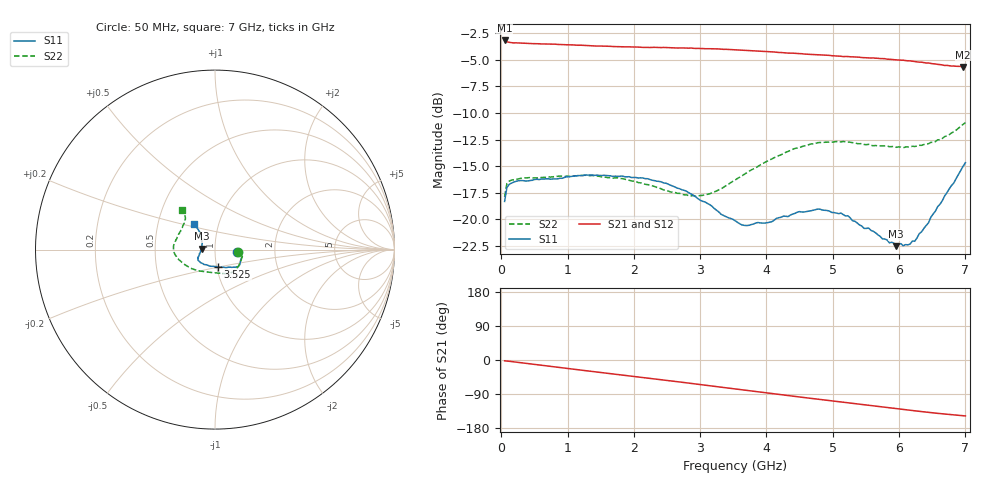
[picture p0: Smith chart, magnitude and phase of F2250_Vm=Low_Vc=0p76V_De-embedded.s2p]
! Integrated Device Technology
! Corporate Headquarters
! 6024 Silver Creek Valley Road
! San Jose, CA 95138  USA
! Phone:  1-408-284-8200
! Toll Free:  1-800-223-1366
! Webpage:  http://www.idt.com/
! Timing and RF Division
! 515 Groton Road, Suite 102
! Westford, MA 01886-6024
! Device:  F2250
! Description: Voltage Variable RF Attenuator
! Frequency:  50.0 -  6000.00 MHz
! Package:  3x3 mm Thin QFN Plastic Package: 16 pin
! Ports:  2 RF, 3 DC
!  Pin  1  = GND
!  Pin  2  = NC
!  Pin  3  = RF1  = Port 1
!  Pin  4  = NC
!  Pin  5  = GND
!  Pin  6  = GND
!  Pin  7  = GND
!  Pin  8  = GND
!  Pin  9  = NC
!  Pin 10  = RF2  = Port 2
!  Pin 11  = NC
!  Pin 12  = GND
!  Pin 13  = GND
!  Pin 14  = VCNTRL
!  Pin 15  = VDD
!  Pin 16  = VMODE
! Vcntrl:  0.760 Volts
! Vmode:  +0.000 Volts
! Vdd:  +3.30  Volts
! Current:  1.159 mA
! Data:  The device was measured on a the F2250 evaluation board which has
!  individual transmission lines to the RF pins.  Data was collected
!  using a calibrated network analyzer.  The evaluation board was
!  de-embedded using a TRL calibration technique.
!  The reference plane is the edge of the package pin.
! Misc:  SN 10
!  Action Tracker AT0258
! Date Measured:  2014-11-26
! Date:  2015-10-15  MJV
! Note:
!  Integrated Device Technology supplies this data as a sample of measured
!  data at the package pin for this product.  Your particular data for this
!  product may vary.
!  Data was taken at 25 degrees C.
!  Integrated Device Technology reserves the right to change this data at anytime.
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# GHz S dB R 50
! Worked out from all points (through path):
!   201 points, 50 MHz to 7 GHz, reference 50 ohm
!   highest |S21| = -3.17 dB at 50 MHz (marker M1); lowest = -5.7 dB at 6.965 GHz (marker M2)
!   group delay of S21, straight-line fit = 59.2 ps
!   lowest |S11| = -22.5 dB at 5.957 GHz (marker M3), VSWR 1.16, Z = 43.1 + j0.442 ohm
!   |S11| at or under -10 dB: start of sweep to end of sweep
!   |S22| runs from -17.9 to -10.9 dB; largest |S21 - S12| = 0.0019
!   S11 on the Smith chart (normalised r, x): 50 MHz: 1.27, -0.03; 3.525 GHz: 1.01, -0.20; 7 GHz: 0.76, +0.23
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0.05  -18.32 -5.0  -3.17 -2.2  -3.17 -2.2  -17.88 -6.2
0.08475  -17.01 -4.3  -3.30 -2.7  -3.30 -2.7  -16.63 -5.3
0.22375  -16.43 -7.2  -3.40 -5.6  -3.39 -5.6  -16.23 -9.7
0.77975  -16.20 -21.4  -3.51 -17.6  -3.51 -17.6  -16.01 -29.9
1.2315  -15.87 -31.3  -3.63 -27.3  -3.64 -27.3  -15.88 -45.0
1.75275  -15.96 -37.2  -3.75 -38.2  -3.75 -38.2  -16.09 -56.9
2.37825  -16.44 -40.6  -3.83 -51.2  -3.83 -51.2  -17.05 -71.3
2.93425  -17.90 -50.1  -3.92 -63.3  -3.91 -63.3  -17.82 -95.9
3.14275  -18.62 -58.8  -3.94 -67.9  -3.95 -67.9  -17.60 -108.8
3.3165  -19.54 -67.7  -3.99 -71.7  -3.99 -71.7  -17.13 -119.1
3.525  -20.13 -81.0  -4.05 -76.3  -4.04 -76.4  -16.32 -130.8
3.7335  -20.57 -97.0  -4.11 -81.0  -4.12 -81.0  -15.50 -140.9
4.04625  -20.28 -116.9  -4.24 -87.8  -4.23 -87.8  -14.43 -154.7
4.39375  -19.51 -134.5  -4.37 -95.3  -4.37 -95.3  -13.42 -166.5
4.7065  -19.15 -145.0  -4.50 -102.0  -4.51 -102.0  -12.91 -174.4
5.22775  -19.67 -156.3  -4.69 -113.0  -4.69 -113.0  -12.73 173.8
5.85325  -22.22 -177.3  -4.95 -126.0  -4.95 -126.0  -13.17 158.1
5.9575  -22.53 176.1  -5.00 -128.2  -5.01 -128.2  -13.23 155.2
6.2355  -22.06 154.1  -5.16 -134.0  -5.16 -134.1  -13.15 145.8
6.61775  -18.58 133.3  -5.44 -141.3  -5.46 -141.4  -12.51 134.0
6.96525  -15.01 129.0  -5.66 -147.1  -5.64 -147.1  -11.07 130.3
7  -14.68 128.6  -5.65 -147.6  -5.65 -147.7  -10.90 129.7
